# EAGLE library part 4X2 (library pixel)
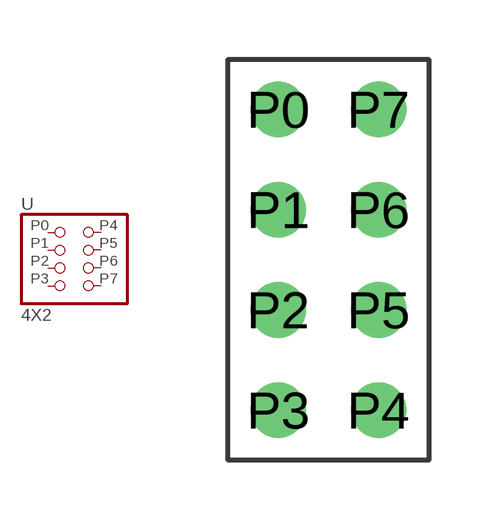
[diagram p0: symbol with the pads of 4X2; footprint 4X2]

Designator prefix -

## 4X2  [4X2]
P0  P0  pas
P1  P1  pas
P2  P2  pas
P3  P3  pas
P4  P4  pas
P5  P5  pas
P6  P6  pas
P7  P7  pas

## Footprint 4X2 (pad centres in mm)
drill 0.9 pad 1.27: P0 -1.27,3.81; P1 -1.27,1.27; P2 -1.27,-1.27; P3 -1.27,-3.81; P4 1.27,-3.81; P5 1.27,-1.27; P6 1.27,1.27; P7 1.27,3.81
